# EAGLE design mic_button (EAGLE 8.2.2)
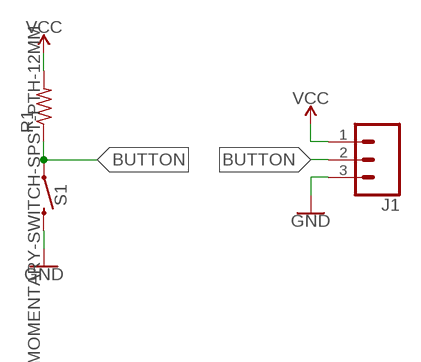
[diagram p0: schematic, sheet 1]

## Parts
J1  CONN_03  [1X03]
R1  R-US_R1206  [R1206]
S1  MOMENTARY-SWITCH-SPST-PTH-12MM  [TACTILE_SWITCH_PTH_12MM]

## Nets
BUTTON: J1.2 R1.1 S1.1
GND: J1.3 S1.3
VCC: J1.1 R1.2

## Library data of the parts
J1 = SparkFun-Connectors:CONN_03: Multi connection point. Often used as Generic Header-pin footprint for 0.1 inch spaced/style header connections On any of the 0.1 inch spaced packages, you can populate with these: Break Away Headers - Straight (PRT-00116) Break Away Male Headers - Right Angle (PRT-00553) Female Headers (PRT-00115)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
R1 = rcl:R-US_: RESISTOR, American symbol
S1 = SparkFun-Switches:MOMENTARY-SWITCH-SPST: Momentary Switch (Pushbutton) - SPST; PROD_ID: SWCH-09185; SF_SKU: COM-09190

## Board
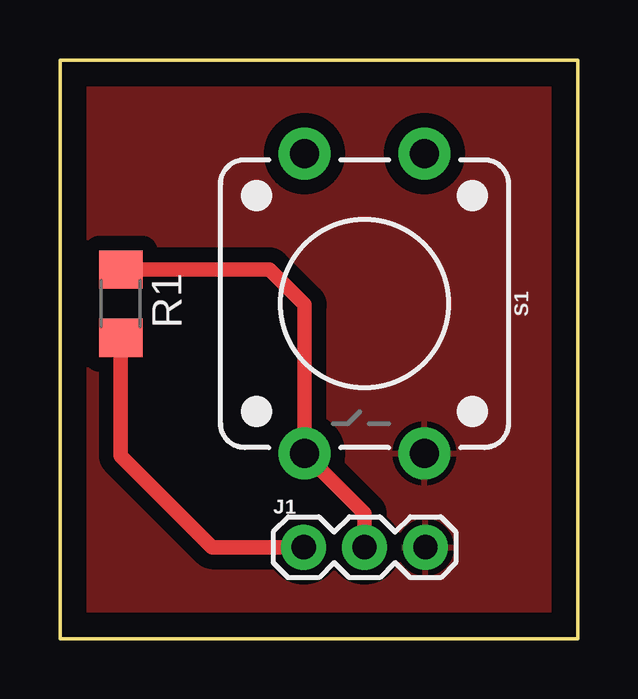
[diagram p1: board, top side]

Size 21.59 x 24.13 mm. Coordinates in mm from the lower left corner, seen from the top.
Outline: 0,0 0,24.13 21.59,24.13 21.59,0 0,0
Copper layers (1*16): Top 0.035mm / dielectric 1.5mm / Bottom 0.035mm
Design rules "default": minimum track width 6mil, minimum drill 0.35mm, track to track 6mil, track to pad 6mil, pad to pad 6mil, via to via 6mil, smd to smd 6mil, copper to edge 40mil, drill to drill 6mil, minimum pad ring 10mil, minimum via ring 8mil, stop-mask expansion 4mil, vias tented up to drill 0mil, thermal gap 10mil

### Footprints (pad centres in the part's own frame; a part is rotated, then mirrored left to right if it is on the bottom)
1X03 = drill 1.016 pad 1.88: 1 0,0; 2 2.54,0; 3 5.08,0
R1206 = smd 1.6 x 1.803: 1 -1.422,0; 2 1.422,0
TACTILE_SWITCH_PTH_12MM = drill 1.2 pad 2.159: 1 6.25,-2.5; 2 -6.25,-2.5; 3 6.25,2.5; 4 -6.25,2.5

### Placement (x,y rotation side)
J1  10.16,3.81 0 top
R1  2.54,13.97 270 top
S1  12.7,13.97 270 top

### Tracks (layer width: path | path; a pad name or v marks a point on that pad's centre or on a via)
BUTTON
  Top 0.61: J1.2 12.7,5.22 S1.1 10.2,13.93 8.74,15.39 R1.1
GND
  pour Top (isolate 0.61): 0,24.13 21.59,24.13 21.59,0 0,0
VCC
  Top 0.61: R1.2 2.54,7.62 6.35,3.81 J1.1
